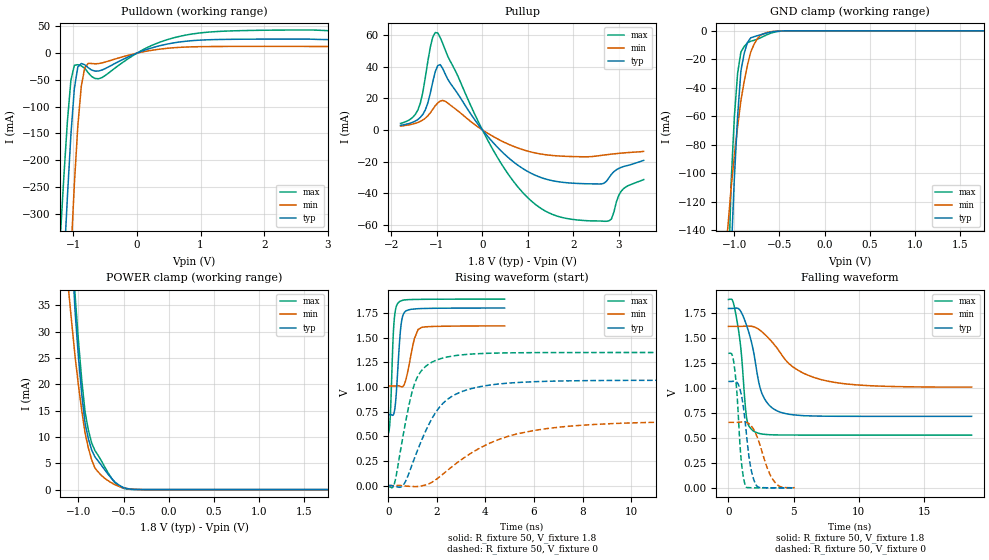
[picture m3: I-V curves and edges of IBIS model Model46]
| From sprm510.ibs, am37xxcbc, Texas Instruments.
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| Model based on original model for BQ18OMAPSMART1HYFBPB_SSBHH
|   Sub model PB_HS10L00_PUPD0_1P8
[model]   Model46
|[Input Load]   PI
|[Output Drive] SC10LB00
|Voltage   1.8V
|Mode   I/O
Model_type   I/O
Polarity   Non-Inverting
Enable   Active-Low
Vinl =  0.63
Vinh =  1.17
Cref =  15pF
Rref =  100.0000M
Vref =  0V
Vmeas =  0.9
C_comp   1.429432p   1.270657p   1.602015p
[Model Spec]
Vinl   0.63   0.567   0.6615
Vinh   1.17   1.053   1.2285
[Temperature Range]   25   125   -40
[Voltage Range]   1.8   1.62   1.89
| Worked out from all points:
|   slope of the pulldown table from 0 to 0.27 V, typ, clamps not added: 24.3 ohm
|   slope of the pullup table from 0 to 0.27 V, typ, clamps not added: 29.7 ohm
|   GND clamp passes 1 mA (typ) near -0.60 V on its own axis
|   POWER clamp passes 1 mA (typ) near -0.56 V on its own axis
|   rising waveform, R_fixture 50, V_fixture 1.8: 20-80 % time 178ps typ, 308ps min, 126ps max; typ from 0.717 V to 1.8 V
|   rising waveform, R_fixture 50, V_fixture 0: 20-80 % time 1.36ns typ, 3ns min, 717ps max; typ from 0 V to 1.07 V
|   falling waveform, R_fixture 50, V_fixture 1.8: 20-80 % time 1.11ns typ, 2.95ns min, 577ps max; typ from 1.8 V to 0.718 V
|   falling waveform, R_fixture 50, V_fixture 0: 20-80 % time 600ps typ, 1.04ns min, 415ps max; typ from 1.07 V to 0 V
[POWER_clamp]
-1.8V     362.5mA    191.4mA    412.8mA
-1.109V   56.69mA    37.71mA    60.38mA
-1.073V   44.6mA     31.22mA    47.8mA
-1.036V   33.44mA    25.04mA    36.59mA
-1V       24.98mA    19.72mA    28.06mA
-963.6mV  18.03mA    14.96mA    20.78mA
-927.3mV  12.59mA    10.77mA    14.74mA
-890.9mV  9.653mA    7.899mA    11.31mA
-818.2mV  6.214mA    4.114mA    7.414mA
-636.4mV  2.183mA    1.307mA    2.238mA
-418.2mV  83.85uA    105.2uA    35.14uA
1.764V    -1.228nA   -79.12nA   -1.453nA
[Pulldown]
-1.8V     -1.718A    -2.61A     -1.406A
-1.2V     -527.4mA   -844.5mA   -339.9mA
-1.145V   -396mA     -683.1mA   -229.1mA
-1.091V   -269mA     -526.7mA   -127.5mA
-1.036V   -153.6mA   -378.9mA   -51.17mA
-981.8mV  -66.34mA   -245.6mA   -22.67mA
-927.3mV  -26mA      -136.2mA   -21.54mA
-872.7mV  -19.34mA   -61.98mA   -23.69mA
-763.6mV  -27.2mA    -19.05mA   -36.72mA
-545.5mV  -31.39mA   -18.17mA   -45.46mA
872.7mV   23.46mA    11.88mA    35.92mA
3.545V    25.34mA    12.51mA    41.58mA
[Pullup]
-1.8V     2.903mA    2.423mA    4.112mA
-1.418V   6.595mA    4.711mA    12.64mA
-1.255V   12.69mA    7.42mA     33.23mA
-1.091V   30.4mA     13mA       58.69mA
-981.8mV  40.63mA    17.02mA    61.3mA
-818.2mV  35.38mA    18.12mA    50.59mA
272.7mV   -9.18mA    -4.728mA   -14.55mA
1.255V    -29.75mA   -15.09mA   -48.97mA
2.564V    -34.17mA   -16.31mA   -57.57mA
2.782V    -30.25mA   -15.5mA    -57.48mA
3.055V    -23.63mA   -14.68mA   -38.61mA
3.545V    -19.25mA   -13.56mA   -31.41mA
[GND_clamp]
-1.8V     -2.82A     -1.192A    -3.165A
-1.073V   -235.7mA   -138.4mA   -192.1mA
-1.036V   -159.5mA   -110.8mA   -107.5mA
-1V       -103.8mA   -87.85mA   -60.67mA
-963.6mV  -60mA      -67.28mA   -29.8mA
-927.3mV  -28.21mA   -49.08mA   -14.9mA
-890.9mV  -15.9mA    -35.48mA   -10.99mA
-854.5mV  -8.138mA   -24.07mA   -8.449mA
-818.2mV  -4.924mA   -14.85mA   -7.266mA
-709.1mV  -2.784mA   -3.064mA   -4.883mA
-563.6mV  -570.2uA   -404.5uA   -1.092mA
1.764V    -11.02pA   583.5nA    3.035nA
[Ramp]
dV/dt_f   0.651474/1.110196n   0.3680192/2.976251n   0.818367/0.5785649n
dV/dt_r  0.6512502/1.36331n   0.4008322/3.024537n   0.82332/0.7192222n
R_load = 50
[Rising Waveform]
R_fixture = 50
V_fixture = 1.8
V_fixture_min = 1.62
V_fixture_max = 1.89
0s        717.3mV    1.009V     528.9mV
81ps      719mV      1.009V     711.8mV
180ps     711.9mV    1.009V     1.404V
234ps     736.7mV    1.009V     1.659V
396ps     1.207V     1.011V     1.849V
522ps     1.627V     1.002V     1.872V
729ps     1.771V     1.081V     1.883V
1.071ns   1.79V      1.488V     1.887V
1.377ns   1.795V     1.603V     1.888V
4.788ns   1.799V     1.618V     1.89V
[Rising Waveform]
R_fixture = 50
V_fixture = 0
V_fixture_min = 0
V_fixture_max = 0
0s        -201.7uV   102.7uV    -10.07mV
243ps     -8.731mV   -231.3uV   13.63mV
666ps     23.42mV    -4.159mV   586.9mV
954ps     196.3mV    -8.604mV   926.7mV
1.143ns   320.9mV    -10.47mV   1.072V
1.728ns   648.9mV    24.58mV    1.242V
2.259ns   835.8mV    118.5mV    1.294V
4.266ns   1.022V     439.3mV    1.342V
6.588ns   1.057V     579.7mV    1.348V
20.6ns    1.067V     655.8mV    1.349V
[Falling Waveform]
R_fixture = 50
V_fixture = 1.8
V_fixture_min = 1.62
V_fixture_max = 1.89
0s        1.8V       1.62V      1.89V
324ps     1.801V     1.62V      1.878V
756ps     1.799V     1.62V      1.597V
1.422ns   1.618V     1.622V     679.4mV
2.016ns   1.3V       1.613V     563mV
2.403ns   1.016V     1.583V     544.8mV
2.772ns   892.7mV    1.542V     537.1mV
4.158ns   752.4mV    1.322V     530.3mV
8.163ns   718.3mV    1.058V     529.8mV
18.66ns   717.6mV    1.011V     529.8mV
[Falling Waveform]
R_fixture = 50
V_fixture = 0
V_fixture_min = 0
V_fixture_max = 0
0s        1.068V     657.3mV    1.349V
279ps     1.068V     657.5mV    1.336V
441ps     1.071V     657.4mV    1.231V
648ps     1.058V     657.5mV    957.5mV
972ps     943.9mV    660.1mV    287.8mV
1.323ns   614.1mV    659mV      15.82mV
1.683ns   222.6mV    631.4mV    1.653mV
2.133ns   26.25mV    534.1mV    281uV
3.51ns    359.7uV    64.64mV    7.9uV
5.085ns   64.41uV    1.629mV    888.9nV
